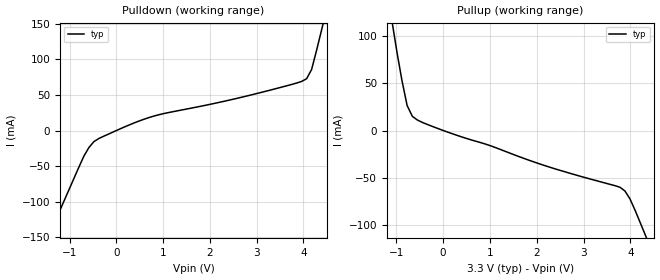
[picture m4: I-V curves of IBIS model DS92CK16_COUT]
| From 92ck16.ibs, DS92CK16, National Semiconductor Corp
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|   CLKout Output  MODEL
[Model]   DS92CK16_COUT
Model_type   Output
| Signals   CLKout0 ~ CLKout5 These signals cannot be TRI-STATED
Vmeas = 1.5V
Cref = 5pF   |Timing specification test load capacitance value
Vref = 0.0   |Timing specification test load voltage; GND
| variable   typ   min   max
C_comp   7.34pF   NA   NA
|   typ   min   max
[Temperature Range]   25.0   NA   NA
[Voltage range]   3.3V   NA   NA
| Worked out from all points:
|   slope of the pulldown table from 0 to 0.495 V, typ, clamps not added: 36.3 ohm
|   slope of the pullup table from 0 to 0.495 V, typ, clamps not added: 58.9 ohm
[Pulldown]
|This output is not a TRI-STATE. It contains the clamp diode values
| measured from -0.8V to 4.5V, then extrapolated to -3.3V and 6.6V
| Voltage   I(typ)   I(min)   I(max)
-3.3V     -426mA     NA         NA
-800mV    -51.53mA   NA         NA
-585mV    -23.86mA   NA         NA
-477mV    -15.5mA    NA         NA
64mV      1.839mA    NA         NA
822mV     20.67mA    NA         NA
2.553V    44.85mA    NA         NA
3.959V    68.98mA    NA         NA
4.067V    72.82mA    NA         NA
4.173V    85.71mA    NA         NA
4.278V    112.3mA    NA         NA
6.6V      733mA      NA         NA
[Pullup]
| Note that the[Pullup]voltage table is referenced to Vcc
| and is calculated using Vtable=Vcc - Vmeasured. This output is
| not a TRI-STATE. It contains the clamp diode values measured
|from -0.8V to 4.5V, then extrapolated to -3.3V and 6.6V
|Voltage  I(typ)   I(min)   I(max)
-3.3V     844.4mA    NA         NA
-1.092V   115.5mA    NA         NA
-882mV    53.38mA    NA         NA
-771mV    26.6mA     NA         NA
-659mV    15.08mA    NA         NA
-550mV    11.12mA    NA         NA
2.045V    -35.16mA   NA         NA
3.777V    -60.19mA   NA         NA
3.885V    -64.2mA    NA         NA
3.992V    -72.6mA    NA         NA
4.102V    -84.75mA   NA         NA
6.6V      -384.8mA   NA         NA
| From SPICE simulations
[Ramp]
|   typ   min   max
dV/dt_r   1.98/1.30n   NA   NA
dV/dt_f   1.98/1.08n   NA   NA
R_load = 1.0M   |the resistive load is a typical scope probe
